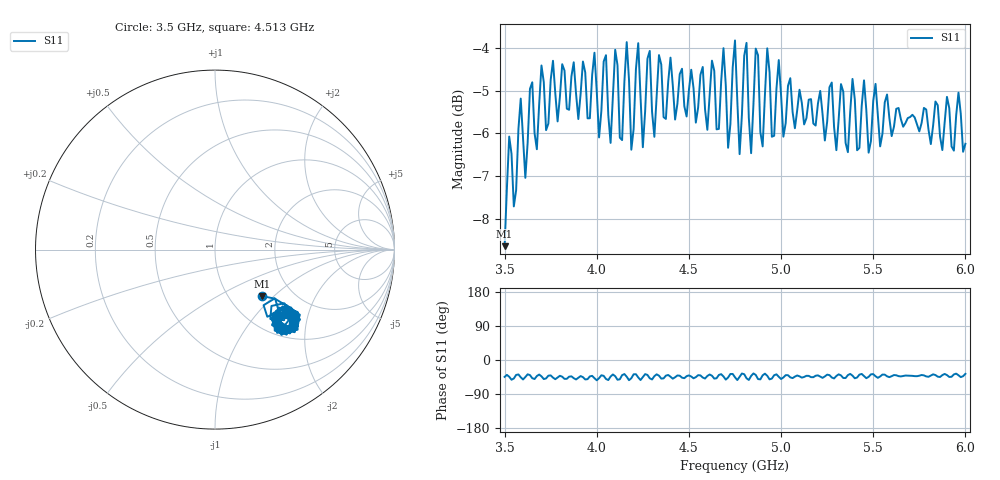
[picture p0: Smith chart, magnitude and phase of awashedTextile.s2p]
!  31/07/2025  11:02:58
! Ref Plane: 0.000 mm
# MHZ S MA R  50
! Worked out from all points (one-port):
!   201 points, 3.5 GHz to 6 GHz, reference 50 ohm
!   lowest |S11| = -8.6 dB at 3.5 GHz (marker M1), VSWR 2.17, Z = 70.8 - j42.5 ohm
!   |S11| at or under -10 dB: nowhere
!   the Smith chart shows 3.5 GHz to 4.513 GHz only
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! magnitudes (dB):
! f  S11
! 3.5 GHz  -8.6
! 3.587 GHz  -5.2
! 3.612 GHz  -7.0
! 3.812 GHz  -4.4
! 4.013 GHz  -6.1
! 4.05 GHz  -4.2
! 4.075 GHz  -6.2
! 4.1 GHz  -4.0
! 4.125 GHz  -6.1
! 4.162 GHz  -3.9
! 4.188 GHz  -6.4
! 4.225 GHz  -3.9
! 4.25 GHz  -6.3
! 4.287 GHz  -4.1
! 4.438 GHz  -5.3
! 4.688 GHz  -4.0
! 4.713 GHz  -6.3
! 4.75 GHz  -3.8
! 4.775 GHz  -6.5
! 4.812 GHz  -3.9
! 4.838 GHz  -6.5
! 4.862 GHz  -4.0
! 4.9 GHz  -6.3
! 4.925 GHz  -4.0
! 5.062 GHz  -5.5
! 5.375 GHz  -5.5
! 5.688 GHz  -5.6
! 6 GHz  -6.2
